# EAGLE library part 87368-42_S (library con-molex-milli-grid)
RECEPTACAL
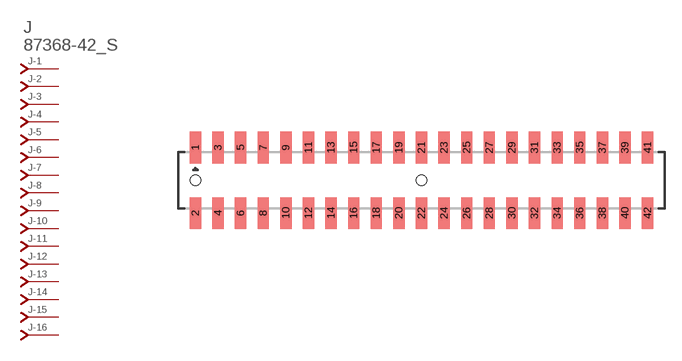
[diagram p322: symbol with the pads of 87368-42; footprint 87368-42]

Designator prefix J; gates -1=J-NV -2=J-N -3=J-N -4=J-N -5=J-N -6=J-N -7=J-N -8=J-N -9=J-N -10=J-N -11=J-N -12=J-N -13=J-N -14=J-N -15=J-N -16=J-N -17=J-N -18=J-N -19=J-N -20=J-N -21=J-N -22=J-N -23=J-N -24=J-N -25=J-N -26=J-N -27=J-N -28=J-N -29=J-N -30=J-N -31=J-N -32=J-N -33=J-N -34=J-N -35=J-N -36=J-N -37=J-N -38=J-N -39=J-N -40=J-N -41=J-N -42=J-N

## 87368-42_S  [87368-42]
1  -1:J  pas
2  -2:J  pas
3  -3:J  pas
4  -4:J  pas
5  -5:J  pas
6  -6:J  pas
7  -7:J  pas
8  -8:J  pas
9  -9:J  pas
10  -10:J  pas
11  -11:J  pas
12  -12:J  pas
13  -13:J  pas
14  -14:J  pas
15  -15:J  pas
16  -16:J  pas
17  -17:J  pas
18  -18:J  pas
19  -19:J  pas
20  -20:J  pas
21  -21:J  pas
22  -22:J  pas
23  -23:J  pas
24  -24:J  pas
25  -25:J  pas
26  -26:J  pas
27  -27:J  pas
28  -28:J  pas
29  -29:J  pas
30  -30:J  pas
31  -31:J  pas
32  -32:J  pas
33  -33:J  pas
34  -34:J  pas
35  -35:J  pas
36  -36:J  pas
37  -37:J  pas
38  -38:J  pas
39  -39:J  pas
40  -40:J  pas
41  -41:J  pas
42  -42:J  pas

## Footprint 87368-42 (pad centres in mm)
RECEPTACAL SMD Dual Row, Side Entry
smd 1 x 2.8: 1 -20,2.9; 2 -20,-2.9; 3 -18,2.9; 4 -18,-2.9; 5 -16,2.9; 6 -16,-2.9; 7 -14,2.9; 8 -14,-2.9; 9 -12,2.9; 10 -12,-2.9; 11 -10,2.9; 12 -10,-2.9; 13 -8,2.9; 14 -8,-2.9; 15 -6,2.9; 16 -6,-2.9; 17 -4,2.9; 18 -4,-2.9; 19 -2,2.9; 20 -2,-2.9; 21 0,2.9; 22 0,-2.9; 23 2,2.9; 24 2,-2.9; 25 4,2.9; 26 4,-2.9; 27 6,2.9; 28 6,-2.9; 29 8,2.9; 30 8,-2.9; 31 10,2.9; 32 10,-2.9; 33 12,2.9; 34 12,-2.9; 35 14,2.9; 36 14,-2.9; 37 16,2.9; 38 16,-2.9; 39 18,2.9; 40 18,-2.9; 41 20,2.9; 42 20,-2.9
hole 0.914 at -20,0
hole 0.914 at 0,0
